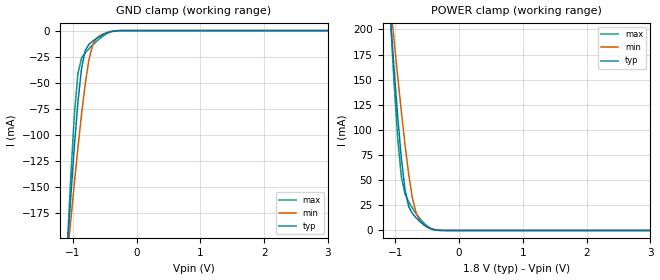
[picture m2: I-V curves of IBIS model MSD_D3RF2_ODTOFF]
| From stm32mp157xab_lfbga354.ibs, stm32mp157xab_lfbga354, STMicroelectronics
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[Model] MSD_D3RF2_ODTOFF
Model_type   Input
C_comp 2.228pF   2.149pF   2.345pF
Vinh = 1.150V
Vinl = 650.000mV
[Model Spec]
Vinh   1.150V   1.100V   1.200V
Vinl   650.000mV   600.000mV   700.000mV
[Temperature Range]   25.000   125.000   -40.000
[Voltage Range]   1.800V   1.700V   1.900V
[GND Clamp Reference]   0.00V   0.00V   0.00V
[POWER Clamp Reference]   1.800V   1.700V   1.900V
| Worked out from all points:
|   GND clamp passes 1 mA (typ) near -0.41 V on its own axis
|   POWER clamp passes 1 mA (typ) near -0.41 V on its own axis
[GND Clamp]
-1.785V   -901.2mA   -688.7mA   -1.21A
-1.094V   -214.6mA   -220.9mA   -215.3mA
-1.036V   -161.8mA   -183.6mA   -143.3mA
-978.8mV  -112.2mA   -147.3mA   -82mA
-921.2mV  -68.48mA   -112.3mA   -40.93mA
-863.6mV  -35.72mA   -79.61mA   -26.14mA
-806.1mV  -18.98mA   -50.61mA   -21.24mA
-748.5mV  -13.21mA   -27.8mA    -17.43mA
-690.9mV  -10.21mA   -13.79mA   -13.87mA
-575.8mV  -5.519mA   -4.737mA   -7.464mA
-287.9mV  -70.53uA   -119uA     -55.71uA
3.57V     33.94nA    572.8nA    3.709nA
[Power Clamp]
-1.77V    882.6mA    689.8mA    1.159A
-1.079V   212.4mA    226.5mA    212.1mA
-1.021V   160.9mA    189.3mA    146.7mA
-963.6mV  112.9mA    152.9mA    90.89mA
-906.1mV  71.15mA    117.8mA    52.89mA
-848.5mV  40.01mA    84.75mA    36.15mA
-790.9mV  23.77mA    55.41mA    28.47mA
-733.3mV  16.96mA    32.2mA     22.3mA
-618.2mV  8.941mA    9.722mA    11.92mA
-503mV    3.409mA    3.507mA    4.442mA
-272.7mV  29.94uA    100.2uA    29.64uA
3.585V    -51.59nA   -928.6nA   -5.521nA
